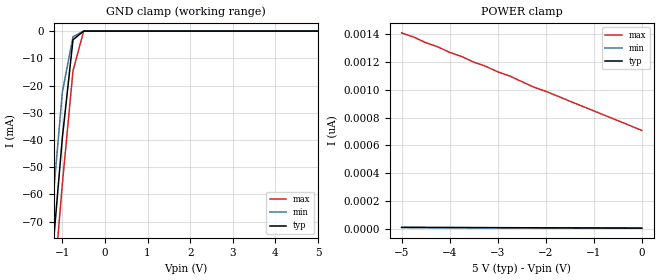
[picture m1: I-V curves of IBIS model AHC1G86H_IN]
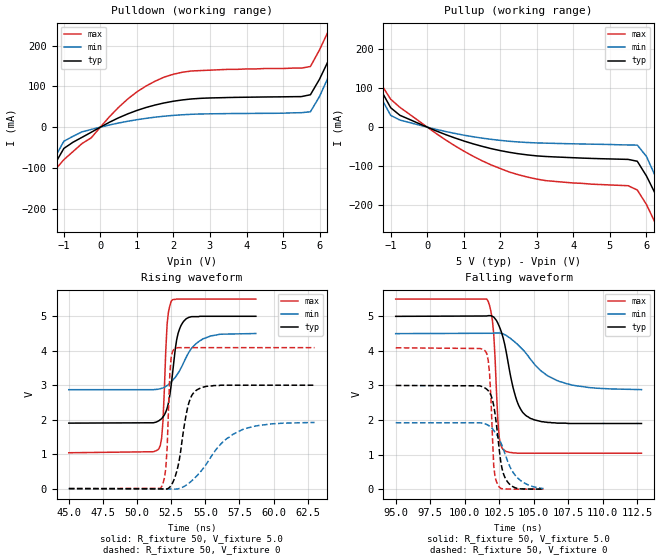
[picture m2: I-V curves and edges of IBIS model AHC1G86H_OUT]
| TEXAS INSTRUMENTS INCORPORATED
| Standard Linear and Logic Group
| IBIS Model of SN74AHC1G86H
| SINGLE 2-INPUT EXCLUSIVE-OR GATE
| CMPAK-5 5-pin (DCK) Package
[IBIS Ver]   2.1
[Comment Char]  |_char
[File name]   ul86_5c.ibs
[File Rev]   2.0
[Date]   April 18, 2000
[Source]   Data created from SPICE simulations at Hitachi,Ltd.
[Notes]   The following is an IBIS List for the AHC1G86H.
|   Please contact sllibis@ti.com with questions and
|   comments concerning SLL IBIS models.
[Disclaimer] Property of Texas Instruments Incorporated.  Unauthorized
   reproduction and/or distribution is strictly prohibited.
   This product is protected under copyright law.
   Created 2000, (C) Copyright 2000, Texas Instruments Inc.,
   All Rights Reserved.
   UNLESS THERE IS A SIGNED, WRITTEN AGREEMENT TO THE
   CONTRARY, TEXAS INSTRUMENTS () IS PROVIDING THE IBIS
   MODELS  AND WITHOUT ANY WARRANTY, EXPRESSED OR
   IMPLIED.  TI assumes no liability for:
   1) the accuracy of the IBIS models provided to your
   company;
   2) the proper functioning of these IBIS Models in your
   design or for any resulting applications; or
   3) infringement of patents, copyrights or intellectual
   property rights resulting from your use of these IBIS
   models.
   TI provides IBIS Models as a service to our customers.
   You and your company shall not distribute, sell or give
   these models to anyone else without prior written
   permission from TI.
   TI reserves the right to make changes to our products or
   to discontinue any semiconductor product or service
   without notice, and advises our customers to obtain the
   latest version of relevant information to verify, before
   placing orders, that the information being relied on is
   current.
   Please be aware that your receipt and use of the IBIS
   information provided shall serve as acceptance of these
   terms and conditions.  If you do not accept these terms,
   you should return or destroy the IBIS models and any
   other accompanying information immediately.
|   Component AHC1G86H
[Component]   AHC1G86H
[Manufacturer]   Hitachi, Ltd.
[Package]
|   typ   min   max
R_pkg   0.090   0.051   0.105
L_pkg   1.500nH   0.940nH   1.700nH
C_pkg   0.170pF   0.110pF   0.360pF
[Pin]   signal_name   model_name   R_pin   L_pin   C_pin
1   A   AHC1G86H_IN   0.098   1.590nH   0.110pF
2   B   AHC1G86H_IN   0.051   0.940nH   0.170pF
3   GND   GND   0.092   1.590nH   0.360pF
4   Y   AHC1G86H_OUT   0.105   1.700nH   0.110pF
5   VCC   POWER   0.104   1.690nH   0.110pF
| Models and submodels in the file (2): AHC1G86H_IN (Input), AHC1G86H_OUT (Output)
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|   Model AHC1G86H_IN
[Model]   AHC1G86H_IN
Model_type  Input
Polarity   Inverting
Vinl = 1.50
Vinh = 3.50
| variable   typ   min   max
C_comp   2.19pF   2.07pF   2.30pF
[Temperature Range]   25   85   -40
[Voltage Range]   5.0   4.5   5.5
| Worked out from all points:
|   GND clamp passes 1 mA (typ) near -0.58 V on its own axis
[GND Clamp]
|   Voltage   I(typ)   I(min)   I(max)
-5V       -823mA     -807mA     -840mA
-1.5V     -133mA     -115mA     -150mA
-1.25V    -85.2mA    -67.5mA    -103mA
-1V       -39.2mA    -22.5mA    -56.2mA
-750mV    -3.18mA    -2.09mA    -14.6mA
-500mV    -11.6uA    -2.99uA    -57.1uA
5V        5.34pA     5pA        708pA
[POWER Clamp]
|   Voltage   I(typ)   I(min)   I(max)
-5V       10.6pA     10pA       1.41nA
-4.75V    10.3pA     9.75pA     1.38nA
-4.5V     10pA       9.5pA      1.34nA
-4.25V    9.78pA     9.25pA     1.31nA
-4V       9.52pA     9pA        1.27nA
-3.75V    9.26pA     8.75pA     1.24nA
-3.5V     9pA        8.5pA      1.2nA
-3.25V    8.74pA     8.25pA     1.17nA
-2.75V    8.21pA     7.75pA     1.1nA
-2.25V    7.69pA     7.25pA     1.02nA
-2V       7.43pA     7pA        990pA
0V        5.34pA     5pA        708pA
|   Model AHC1G86H_OUT
[Model]   AHC1G86H_OUT
Model_type  Output
Polarity   Inverting
Vmeas = 2.5
Cref = 15pf
| variable   typ   min   max
C_comp   4.52pF   4.32pF   4.72pF
[Temperature Range]   25   85   -40
[Voltage Range]   5.0   4.5   5.5
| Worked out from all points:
|   slope of the pulldown table from 0 to 0.75 V, typ, clamps not added: 23 ohm
|   slope of the pullup table from 0 to 0.75 V, typ, clamps not added: 27.3 ohm
|   rising waveform, R_fixture 50, V_fixture 5.0: 20-80 % time 620ps typ, 1.52ns min, 288ps max; typ from 1.9 V to 5 V
|   falling waveform, R_fixture 50, V_fixture 5.0: 20-80 % time 1.03ns typ, 2.52ns min, 339ps max; typ from 5 V to 1.9 V
|   falling waveform, R_fixture 50, V_fixture 0: 20-80 % time 591ps typ, 1.3ns min, 275ps max; typ from 3 V to 0.001 V
|   rising waveform, R_fixture 50, V_fixture 0: 20-80 % time 766ps typ, 2.48ns min, 252ps max; typ from 0 V to 3 V
[Pulldown]
|   Voltage   I(typ)   I(min)   I(max)
-5V       -826mA     -810mA     -842mA
-2.25V    -282mA     -267mA     -299mA
-2V       -234mA     -219mA     -250mA
-1.25V    -91.3mA    -75.2mA    -106mA
-1V       -52.3mA    -34.7mA    -80mA
750mV     32.6mA     14.5mA     69.2mA
1.75V     59.5mA     26.9mA     123mA
5.75V     79.6mA     37.8mA     149mA
6.25V     165mA      125mA      238mA
6.75V     261mA      217mA      336mA
7V        310mA      265mA      385mA
10V       906mA      861mA      980mA
[Pullup]
|   Voltage   I(typ)   I(min)   I(max)
-5V       828mA      811mA      845mA
-2.25V    284mA      267mA      301mA
-2V       235mA      218mA      252mA
-1V       49.6mA     30.1mA     71.4mA
750mV     -27.5mA    -16mA      -47.4mA
2.25V     -64.5mA    -36.2mA    -115mA
5.75V     -87.4mA    -46mA      -161mA
6V        -125mA     -75mA      -198mA
6.25V     -172mA     -127mA     -247mA
6.75V     -269mA     -224mA     -345mA
7V        -318mA     -273mA     -395mA
10V       -917mA     -874mA     -991mA
[Ramp]
| variable   typ   min   max
dV/dt_r   1.80E+00/7.60E-10   1.15E+00/2.48E-09   2.45E+00/2.50E-10
dV/dt_f   1.86E+00/1.03E-09   9.74E-01/2.51E-09   2.68E+00/3.30E-10
R_load = 50
[Rising Waveform]
R_fixture = 50
V_fixture = 5.0
V_fixture_min = 4.5
V_fixture_max = 5.5
|   Time   V(typ)   V(min)   V(max)
45ns      1.9V       2.87V      1.04V
51.5ns    1.95V      2.88V      1.12V
51.8ns    2.03V      2.91V      1.47V
51.9ns    2.08V      2.92V      1.98V
52.2ns    2.33V      2.99V      4.78V
52.5ns    3.01V      3.1V       5.44V
53ns      4.5V       3.35V      5.5V
53.6ns    4.93V      3.81V      5.5V
55.4ns    5V         4.43V      5.5V
58.7ns    5V         4.5V       5.5V
[Falling Waveform]
R_fixture = 50
V_fixture = 5.0
V_fixture_min = 4.5
V_fixture_max = 5.5
|   Time   V(typ)   V(min)   V(max)
95ns      5V         4.5V       5.5V
101.6ns   5.01V      4.51V      5.5V
102ns     5V         4.51V      4.9V
102.1ns   4.98V      4.51V      4.49V
102.5ns   4.71V      4.52V      1.49V
102.8ns   4.35V      4.49V      1.14V
103.7ns   2.65V      4.23V      1.05V
104.7ns   2.06V      3.79V      1.04V
107.3ns   1.91V      3.06V      1.04V
112.8ns   1.9V       2.88V      1.04V
[Falling Waveform]
R_fixture = 50
V_fixture = 0
|   Time   V(typ)   V(min)   V(max)
95ns      3V         1.92V      4.09V
101.4ns   2.94V      1.9V       4.03V
101.6ns   2.89V      1.87V      3.92V
101.8ns   2.79V      1.82V      3.34V
102.1ns   2.42V      1.7V       680mV
102.4ns   1.51V      1.52V      117mV
102.7ns   598mV      1.26V      12.3mV
103.2ns   163mV      715mV      3.4mV
104.2ns   7mV        206mV      277uV
105.7ns   1.31mV     18.3mV     -45uV
[Rising Waveform]
R_fixture = 50
V_fixture = 0
|   Time   V(typ)   V(min)   V(max)
45ns      0V         0V         0V
51.8ns    -11mV      -4.36mV    58.4mV
52.1ns    -16.5mV    -7.89mV    575mV
52.4ns    44.2mV     -11.6mV    3.35V
52.5ns    95.5mV     -12.7mV    3.83V
52.8ns    363mV      -15.1mV    4.07V
53.7ns    2.35V      128mV      4.09V
54.4ns    2.87V      380mV      4.09V
57.7ns    3V         1.71V      4.09V
63ns      3V         1.92V      4.09V
